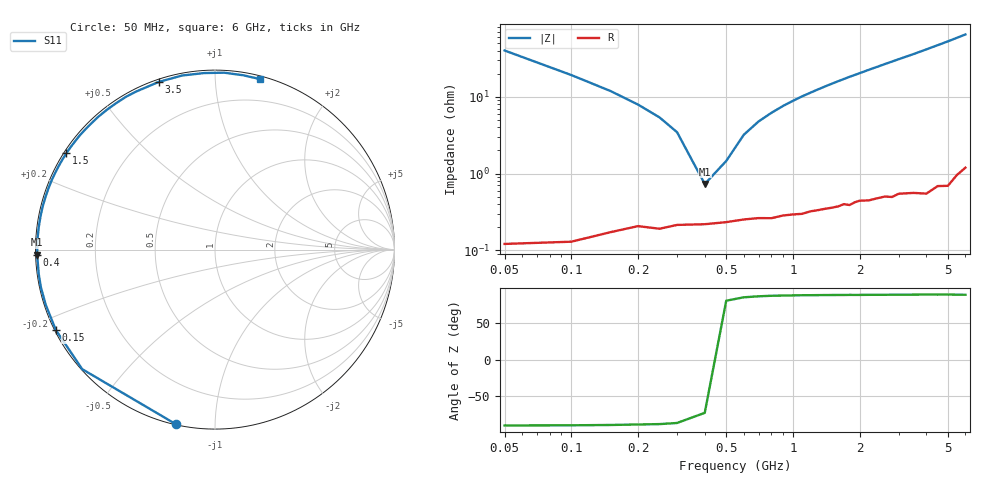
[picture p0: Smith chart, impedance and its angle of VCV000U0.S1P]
! Infineon Technologies  Discrete & RF Semiconductors
! BBY 56-03
! Si Tuning Diode in SOD323
! VR = 0 V
! S-Parameters:  June  1999
# GHz  S  MA  R  50
!  f  S11
! GHz  MAG  ANG
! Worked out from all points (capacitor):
!   34 points, 50 MHz to 6 GHz, reference 50 ohm
!   read as one part to ground: C = 78.4 pF near 50 MHz
!   lowest |Z| = 732 mohm at 400 MHz (marker M1)
!   series resonance near 432.6 MHz, so ESL is about 1.7 nH
!   S11 on the Smith chart (normalised r, x): 50 MHz: 0.00, -0.80; 150 MHz: 0.00, -0.24; 400 MHz: 0.00, -0.01; 1.5 GHz: 0.01, +0.30; 3.5 GHz: 0.01, +0.72; 6 GHz: 0.02, +1.30
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0.05  0.997 -102.6
0.1  0.9955 -138.0
0.15  0.9935 -153.2
0.2  0.992 -162.0
0.25  0.9925 -167.7
0.3  0.9915 -172.1
0.4  0.9913 -178.4
0.5  0.9907 176.7
0.6  0.99 172.7
0.7  0.9896 169.1
0.8  0.9897 165.9
0.9  0.9889 162.8
1.1  0.9886 157.1
1.3  0.9875 151.9
1.5  0.9869 147.0
1.6  0.9865 144.6
1.8  0.9863 140.0
2  0.9849 135.8
2.2  0.9852 131.6
2.4  0.9848 127.7
2.6  0.9845 123.8
3  0.9843 116.6
3.5  0.9854 108.5
4  0.9871 100.7
4.5  0.9855 93.5
5  0.9869 87.0
5.5  0.984 80.8
6  0.9824 75.3
